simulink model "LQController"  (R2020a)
settings: Solver=VariableStepAuto  StartTime=0.0  StopTime=10.0  RelTol=1e-3
InitFcn:
  | initParams
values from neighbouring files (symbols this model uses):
  K = 10    [initParams.m]
  x0 = [0.2;0.1]    [initParams.m]

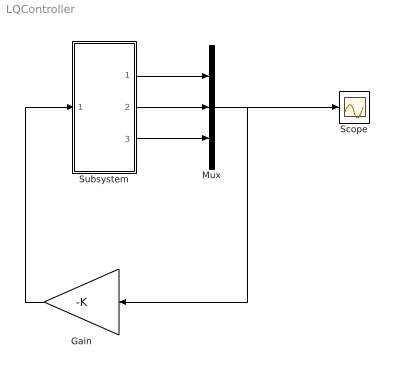
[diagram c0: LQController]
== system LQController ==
  Gain : Gain  Gain=-K  Multiplication=Matrix(K*u) (u vector)
  Mux : Mux  Inputs=3
  Scope : Scope
  Subsystem : Subsystem
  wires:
  Subsystem/2(x2) -> Mux/2
  Subsystem/1(x1) -> Mux/1
  Subsystem/3(x3) -> Mux/3
  Mux/1 -> Scope/1, Gain/1
  Gain/1 -> Subsystem/1(u)

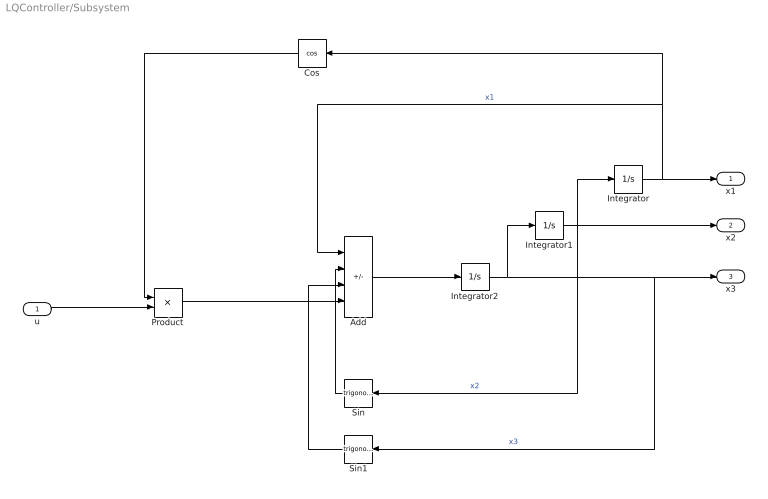
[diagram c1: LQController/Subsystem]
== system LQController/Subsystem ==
  u : Inport
  Add : Sum  Inputs=---+
  Cos : Trigonometry  Operator=cos
  Integrator : Integrator  InitialCondition=x0(1)
  Integrator1 : Integrator  InitialCondition=x0(1)
  Integrator2 : Integrator  InitialCondition=x0(3)
  Product : Product
  Sin : Trigonometry
  Sin1 : Trigonometry
  x1 : Outport
  x2 : Outport  Port=2
  x3 : Outport  Port=3
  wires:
  u/1 -> Product/2
  Cos/1 -> Product/1
  Integrator/1 -> x1/1, Add/1, Cos/1  "x1"
  Integrator2/1 -> x3/1, Sin1/1, Integrator1/1  "x3"
  Sin/1 -> Add/2
  Sin1/1 -> Add/3
  Add/1 -> Integrator2/1
  Integrator1/1 -> x2/1, Sin/1, Integrator/1  "x2"
  Product/1 -> Add/4
